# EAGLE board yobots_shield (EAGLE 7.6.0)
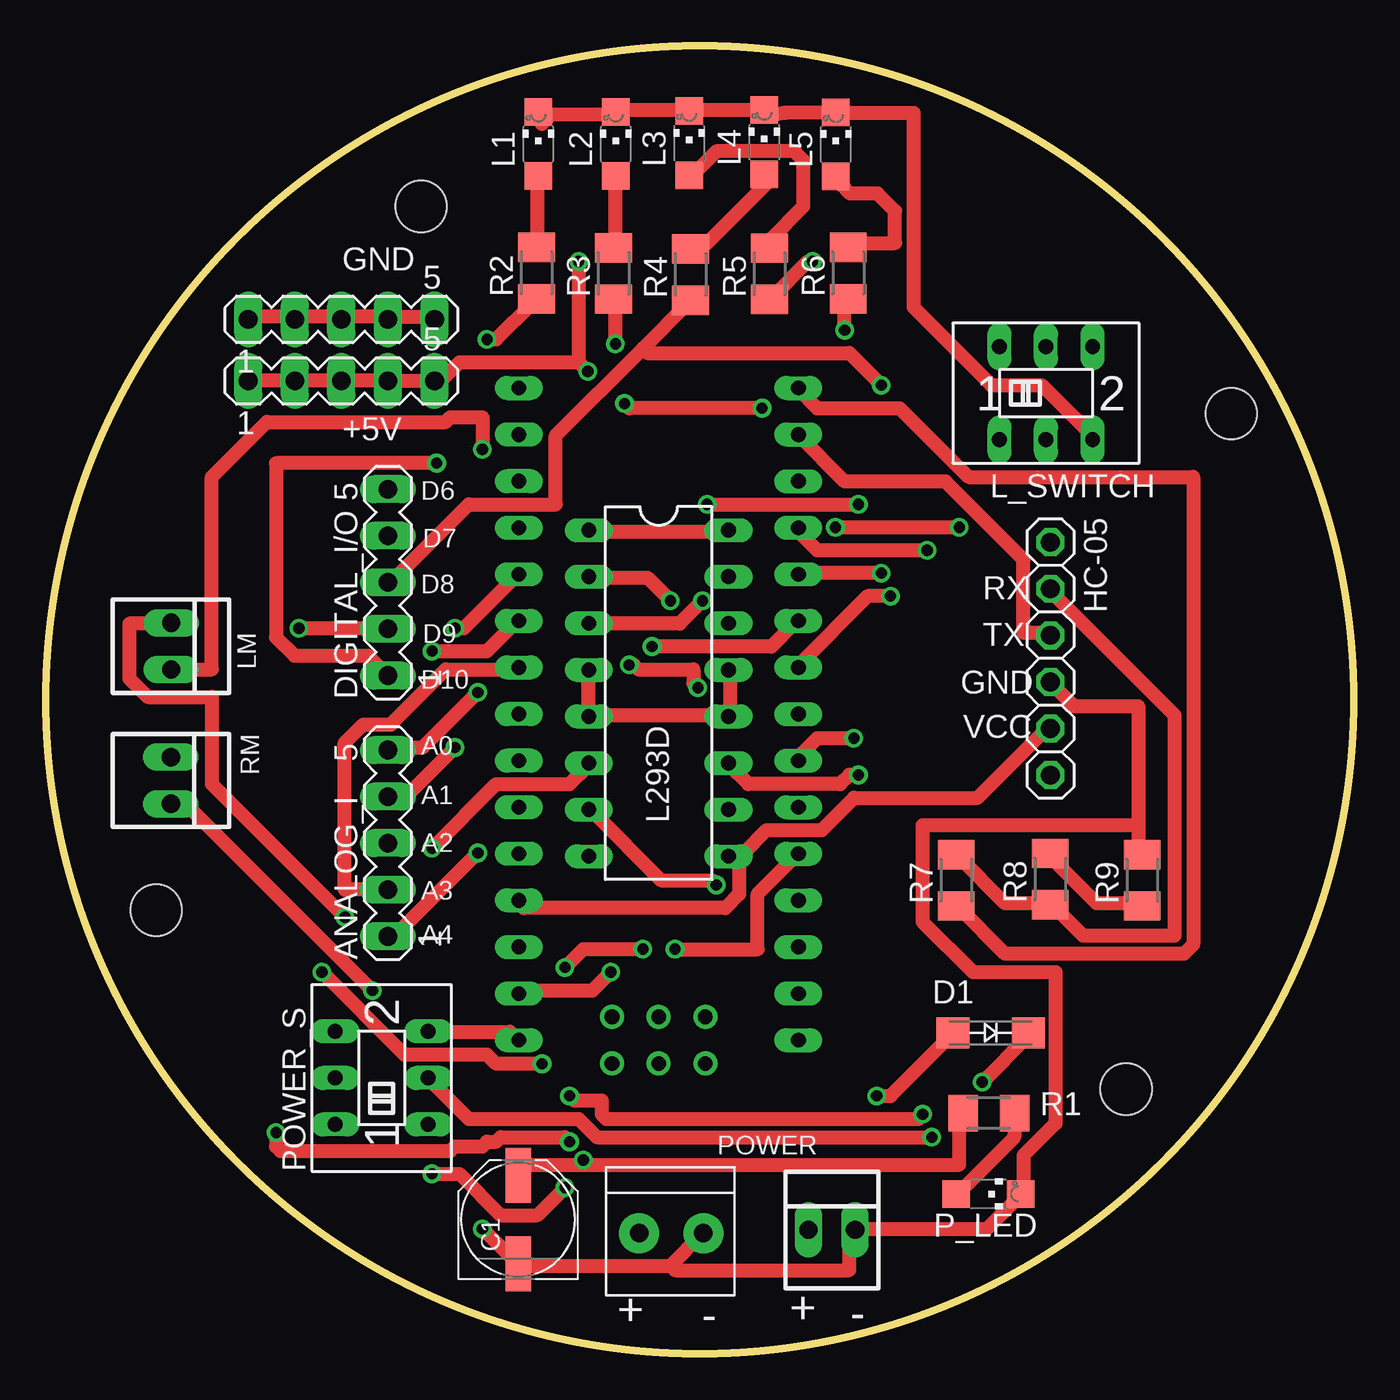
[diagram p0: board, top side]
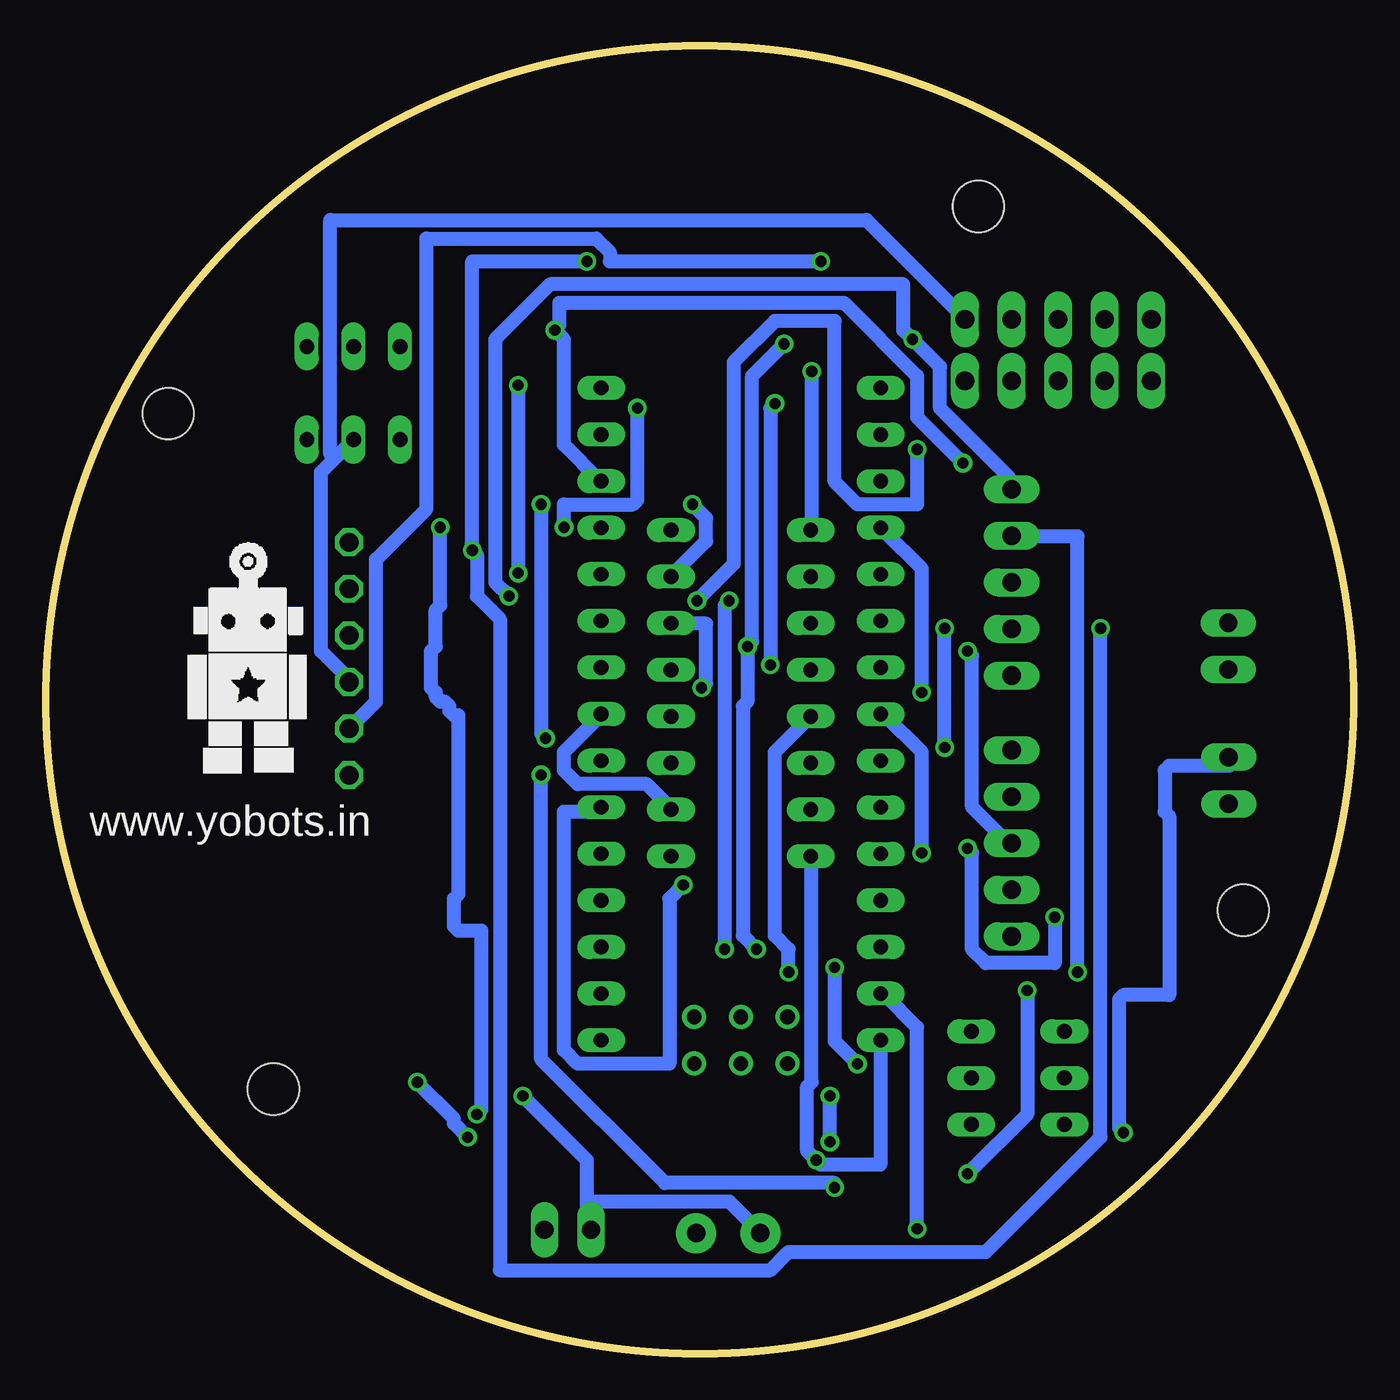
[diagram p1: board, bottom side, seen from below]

Size 71.3 x 71.3 mm. Coordinates in mm from the lower left corner, seen from the top.
Outline: circle at 35.65,35.65 radius 35.65
Copper layers (1*16): Top 0.035mm / dielectric 1.5mm / Bottom 0.035mm
Design rules "default": minimum track width 10mil, minimum drill 24mil, track to track 8mil, track to pad 8mil, pad to pad 8mil, via to via 8mil, smd to smd 8mil, copper to edge 40mil, drill to drill 8mil, minimum pad ring 10mil, minimum via ring 8mil, stop-mask expansion 4mil, vias tented up to drill 0mil, thermal gap 10mil
Net classes: 0 default: width 0.762 mm
Holes 2.8 mm at 20.45,62.55 64.63,51.25 58.9,14.42 6.01,24.18

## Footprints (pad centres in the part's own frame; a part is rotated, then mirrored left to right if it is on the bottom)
MA05-1 = drill 1.016 long: 1 -5.08,0; 2 -2.54,0; 3 0,0; 4 2.54,0; 5 5.08,0
PANASONIC_D = smd 3 x 1.4: + 2.4,0; - -2.4,0
SMA-DO214AC = smd 1.8 x 1.7: A -2.05,0; K 2.05,0
1X06 = drill 1.016 octagon: 1 -6.35,0; 2 -3.81,0; 3 -1.27,0; 4 1.27,0; 5 3.81,0; 6 6.35,0
1X2-3.5MM = drill 1 pad 2.184: 1 1.8,0; 2 -1.7,0
CHIPLED_1206 = smd 1.5 x 1.5: A 0,-1.75; C 0,1.75
DIL16 = drill 0.813 long: 1 -8.89,-3.81; 2 -6.35,-3.81; 3 -3.81,-3.81; 4 -1.27,-3.81; 5 1.27,-3.81; 6 3.81,-3.81; 7 6.35,-3.81; 8 8.89,-3.81; 9 8.89,3.81; 10 6.35,3.81; 11 3.81,3.81; 12 1.27,3.81; 13 -1.27,3.81; 14 -3.81,3.81; 15 -6.35,3.81; 16 -8.89,3.81
A68-A31 = drill 0.813 long: 1 -2.54,-2.54; 2 0,-2.54; 3 2.54,-2.54; 4 -2.54,2.54; 5 0,2.54; 6 2.54,2.54
22-23-2021 = drill 1 long: 1 -1.27,0; 2 1.27,0
M1206 = smd 1.6 x 2: 1 -1.4,0; 2 1.4,0
NANO = drill 0.8 long: 3.3V -10.16,24.13; 5V -10.16,-1.27; A0 -10.16,19.05; A1 -10.16,16.51; A2 -10.16,13.97; A3 -10.16,11.43; A4 -10.16,8.89; A5 -10.16,6.35; A6 -10.16,3.81; A7 -10.16,1.27; AREF -10.16,21.59; D2 5.08,1.27; D3 5.08,3.81; D4 5.08,6.35; D5 5.08,8.89; D6 5.08,11.43; D7 5.08,13.97; D8 5.08,16.51; D9 5.08,19.05; D10 5.08,21.59; D11 5.08,24.13; D12 5.08,26.67; D13 -10.16,26.67; GND -10.16,-6.35; GND1 5.08,-1.27; RAW -10.16,-8.89; RST -10.16,-3.81; RST1 5.08,-3.81; RX1 5.08,-6.35; TX0 5.08,-8.89 | drill 0.8: ICSP1 -5.08,-10.16; ICSP2 -5.08,-7.62; ICSP3 -2.54,-10.16; ICSP4 -2.54,-7.62; ICSP5 0,-10.16; ICSP6 0,-7.62

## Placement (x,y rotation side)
+5V  [MA05-1]  16.11,53.03 0 top
ANALOG_I  [MA05-1]  18.65,27.83 90 top
C1  [PANASONIC_D]  25.75,7.31 90 top
D1  [SMA-DO214AC]  51.51,17.49 0 top
DIGITAL_I/O  [MA05-1]  18.65,42.05 90 top
GND  [MA05-1]  16.11,56.39 0 top
HC-05  [1X06]  54.77,37.89 270 top
J1  [1X2-3.5MM]  34.15,6.57 180 top
L1  [CHIPLED_1206]  26.85,65.95 0 top
L2  [CHIPLED_1206]  31.07,65.95 0 top
L3  [CHIPLED_1206]  35.07,65.99 0 top
L4  [CHIPLED_1206]  39.17,66.05 0 top
L5  [CHIPLED_1206]  43.07,65.93 0 top
L293D  L293D  [DIL16]  33.41,36.01 270 top
L_SWITCH  [A68-A31]  54.53,52.37 0 top
LM  [22-23-2021]  6.83,38.57 270 top
P_LED  [CHIPLED_1206]  51.39,8.71 270 top
POWER  [22-23-2021]  42.85,6.75 0 top
POWER_S  [A68-A31]  18.31,15.03 90 top
R1  [M1206]  51.41,13.11 0 top
R2  [M1206]  26.75,58.91 90 top
R3  [M1206]  30.95,58.89 90 top
R4  [M1206]  35.15,58.83 90 top
R5  [M1206]  39.45,58.87 90 top
R6  [M1206]  43.75,58.91 90 top
R7  [M1206]  49.63,25.81 90 top
R8  [M1206]  54.75,25.87 90 top
R9  [M1206]  59.77,25.81 90 top
RM  [22-23-2021]  6.81,31.25 270 top
U$1  NANO  [NANO]  35.95,25.98 0 top

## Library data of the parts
+5V ANALOG_I DIGITAL_I/O GND = con-lstb; OC_FARNELL: unknown; OC_NEWARK: unknown
C1 = rcl
D1 = diode
HC-05 J1 L1-L5 P_LED R1-R9 = adafruit
L293D = st-microelectronics; MPN: L293D; OC_FARNELL: 9589619; OC_NEWARK: 56P8249
L_SWITCH POWER_S = switch
LM POWER RM = con-molex; MF: MOLEX; MPN: 22-23-2021; OC_FARNELL: 1462926; OC_NEWARK: 25C3832
U$1 = Arduino-clone

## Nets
5V: +5V.1 +5V.2 +5V.3 +5V.4 +5V.5 HC-05.5 L293D.1 L293D.9 L293D.16 U$1.5V
+9V: C1.+ L293D.8 POWER_S.3 R1.1 U$1.RAW
A0: ANALOG_I.5 U$1.A0
A1: ANALOG_I.4 U$1.A1
A2: ANALOG_I.3 U$1.A2
A3: ANALOG_I.2 U$1.A3
A4: ANALOG_I.1 U$1.A4
D2: L293D.2 U$1.D2
D3: L293D.7 U$1.D3
D4: L293D.15 U$1.D4
D5: L293D.10 U$1.D5
D6: DIGITAL_I/O.5 R2.1 U$1.D6
D7: DIGITAL_I/O.4 R3.1 U$1.D7
D8: DIGITAL_I/O.3 R4.1 U$1.D8
D9: DIGITAL_I/O.2 R5.1 U$1.D9
D10: DIGITAL_I/O.1 R6.1 U$1.D10
GND: C1.- GND.1 GND.2 GND.3 GND.4 GND.5 HC-05.4 J1.2 L293D.4 L293D.5 L293D.12 L293D.13 L_SWITCH.2 P_LED.C POWER.2 R9.2 U$1.GND
M1: L293D.3 LM.2
M2: L293D.6 LM.1
M3: L293D.14 RM.1
M4: L293D.11 RM.2
N$1: D1.A J1.1 POWER.1
N$2: P_LED.A R1.2
N$3: D1.K POWER_S.2
N$4: L1.A R2.2
N$5: L2.A R3.2
N$6: L4.A R4.2
N$7: HC-05.2 R7.2 R8.1
N$8: R8.2 R9.1
N$12: L3.A R5.2
N$13: L5.A R6.2
N$15: L1.C L2.C L3.C L4.C L5.C L_SWITCH.3
RX: HC-05.3 U$1.D11
TX: R7.1 U$1.D12

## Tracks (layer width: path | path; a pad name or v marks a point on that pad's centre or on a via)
5V  (via drill 0.61)
  Top 0.762: L293D.1 29.8,44.8 37.05,44.8 L293D.16 | +5V.1 11.05,53.05 13.55,53.05 +5V.2 13.8,53.05 15.8,53.05 +5V.3 16.3,53.05 18.55,53.05 +5V.4 18.8,53.05 21.05,53.05 +5V.5 21.55,53.05 22.55,54.05 29.05,54.05 | 29.05,54.05 v29.55,53.55 | U$1.5V 25.8,24.55 26.05,24.3 37.05,24.3 37.8,25.05 37.8,27.05 37.3,27.05 L293D.9 38.05,27.3 39.3,28.55 42.3,28.55 44.05,30.3 50.8,30.3 54.55,34.05 HC-05.5 | v29.05,59.55 29.05,54.05
  Bottom 0.762: v29.55,53.55 29.55,45.05 L293D.1 | v29.05,59.55 40.55,59.55 40.55,60.05 41.3,60.8 50.55,60.8 50.55,46.05 53.3,43.3 53.3,35.55 HC-05.5
+9V  (via drill 0.61)
  Top 0.762: U$1.RAW 25.55,17.3 25.3,17.55 21.05,17.55 POWER_S.3 | 29.3,10.3 26.3,10.3 25.8,9.8 C1.+ | 29.3,10.3 49.8,10.3 49.8,13.05 R1.1 | v29.3,10.55 29.3,10.3
  Bottom 0.762: L293D.8 29.55,27.05 29.55,14.8 29.8,14.55 29.8,11.05 v29.3,10.55 29.05,10.3 25.8,10.3 25.8,17.05 U$1.RAW
A0  (via drill 0.61)
  Top 0.762: v23.55,36.05 20.55,33.05 18.8,33.05 ANALOG_I.5
  Bottom 0.762: v23.55,36.05 23.55,42.8 25.55,44.8 U$1.A0
A1  (via drill 0.61)
  Top 0.762: v22.3,39.55 22.8,39.55 25.55,42.3 U$1.A1 | v22.3,33.05 19.8,30.55 18.8,30.55 ANALOG_I.4
  Bottom 0.762: v22.3,33.05 v22.3,39.55
A2  (via drill 0.61)
  Top 0.762: v21.05,38.3 24.05,38.3 25.55,39.8 U$1.A2
  Bottom 0.762: v21.05,38.3 20.8,38.05 20.8,29.8 18.8,27.8 ANALOG_I.3
A3
  Top 0.762: U$1.A3 25.55,37.3 21.8,37.3 18.8,34.3 17.3,34.3 16.3,33.3 16.3,25.3 18.55,25.3 ANALOG_I.2
A4  (via drill 0.61)
  Top 0.762: v23.55,27.3 19.05,22.8 18.8,22.8 ANALOG_I.1
  Bottom 0.762: v23.55,27.3 23.55,32.8 25.55,34.8 U$1.A4
D2  (via drill 0.61)
  Top 0.762: v34.3,22.05 38.8,22.05 38.8,25.05 40.8,27.05 U$1.D2 | v34.05,41.05 32.8,42.3 29.8,42.3 L293D.2
  Bottom 0.762: v34.3,22.05 34.3,40.8 v34.05,41.05
D3  (via drill 0.61)
  Top 0.762: v36.55,25.55 36.3,25.8 33.55,25.8 29.8,29.55 L293D.7
  Bottom 0.762: v36.55,25.55 37.3,24.8 37.3,15.8 42.3,15.8 43.05,16.55 43.05,29.55 41.05,29.55 U$1.D3
D4  (via drill 0.61)
  Top 0.762: v44.05,33.55 42.05,33.55 41.05,32.55 U$1.D4 | v36.05,46.3 v44.3,46.3
  Bottom 0.762: v44.05,33.55 44.3,33.8 v44.3,46.3 | v36.05,46.3 35.3,45.55 35.3,44.3 37.05,42.55 L293D.15
D5
  Bottom 0.762: U$1.D5 41.05,34.8 43.05,32.8 43.05,31.8 42.3,31.05 38.55,31.05 37.3,29.8 L293D.10
D6  (via drill 0.61)
  Top 0.762: v24.05,55.3 24.55,55.3 26.55,57.3 R2.1 | v46.05,41.3 44.8,41.3 41.05,37.55 U$1.D6
  Bottom 0.762: DIGITAL_I/O.5 18.8,47.3 18.8,47.8 22.55,51.55 22.55,53.8 v24.05,55.3 24.55,55.8 24.55,58.3 43.8,58.3 46.8,55.3 46.8,42.05 v46.05,41.3
D7  (via drill 0.61)
  Top 0.762: v31.05,55.05 31.05,57.3 R3.1 | v33.05,38.55 39.55,38.55 40.8,39.8 U$1.D7 | v15.05,20.8 19.55,16.3 24.05,16.3 24.55,15.8 v27.05,15.8 | v28.3,21.05 29.3,22.05 v32.55,22.05
  Bottom 0.762: v31.05,55.05 32.8,53.3 32.8,38.8 v33.05,38.55 33.05,35.55 33.3,35.3 33.3,22.8 v32.55,22.05 | v15.05,20.8 15.05,44.55 18.55,44.55 DIGITAL_I/O.4 | v27.05,15.8 28.3,17.05 v28.3,21.05
D8  (via drill 0.61)
  Top 0.762: 32.55,54.8 27.8,50.05 27.8,46.3 23.05,46.3 18.8,42.05 DIGITAL_I/O.3 | 32.55,54.8 35.05,57.3 R4.1 | v45.55,42.55 41.05,42.55 U$1.D8 | v45.55,52.8 43.8,54.55 32.8,54.55 32.55,54.8
  Bottom 0.762: v45.55,52.8 v45.55,42.55
D9  (via drill 0.61)
  Top 0.762: v41.8,59.55 41.55,59.55 39.55,57.55 R5.1 | v48.05,43.8 42.05,43.8 41.05,44.8 U$1.D9 | v13.8,39.55 18.55,39.55 DIGITAL_I/O.2
  Bottom 0.762: v41.8,59.55 48.05,59.55 v48.05,43.8 47.8,43.55 47.8,41.3 46.55,40.05 46.55,4.55 31.8,4.55 30.8,5.55 20.05,5.55 13.8,11.8 v13.8,39.55
D10  (via drill 0.61)
  Top 0.762: v43.55,55.8 43.55,57.3 R6.1 | v21.3,48.55 12.55,48.55 12.55,39.05 13.55,38.05 17.55,38.05 18.55,37.05 DIGITAL_I/O.1
  Bottom 0.762: U$1.D10 41.05,47.55 43.05,49.55 43.05,55.3 v43.55,55.8 43.3,56.05 43.3,57.3 27.8,57.3 23.8,53.3 23.8,51.05 v21.3,48.55
GND  (via drill 0.61)
  Top 0.762: L293D.4 29.55,37.05 29.55,34.8 L293D.5 29.8,34.8 37.05,34.8 L293D.12 37.3,34.8 37.3,37.05 L293D.13 | v23.8,6.8 25.55,5.05 C1.- 26.05,4.8 34.05,4.8 | 34.05,4.8 35.8,6.55 J1.2 | 34.05,4.8 34.3,4.55 43.8,4.55 43.8,6.55 POWER.2 44.3,6.8 51.3,6.8 53.05,8.55 P_LED.C 53.3,9.05 53.3,10.8 55.05,12.55 55.05,20.8 50.55,20.8 47.8,23.55 47.8,28.8 59.55,28.8 | v30.8,20.8 29.8,19.8 25.8,19.8 U$1.GND | GND.1 11.05,56.55 13.55,56.55 GND.2 13.8,56.55 15.8,56.55 GND.3 16.3,56.55 18.55,56.55 GND.4 18.8,56.55 21.05,56.55 GND.5 | 59.55,28.8 59.55,35.3 56.05,35.3 54.8,36.55 HC-05.4 | 59.55,28.8 59.55,27.3 R9.2
  Bottom 0.762: v23.8,6.8 23.8,17.8 25.55,19.55 U$1.GND | v30.8,20.8 30.8,22.05 31.55,22.8 31.55,32.8 29.8,34.55 L293D.5 | 55.55,48.8 56.3,48.05 56.3,38.3 54.8,36.8 HC-05.4 | 55.55,48.8 54.55,49.8 L_SWITCH.2 | GND.5 21.3,56.55 26.55,61.8 55.8,61.8 55.8,49.05 55.55,48.8
M1  (via drill 0.61)
  Top 0.762: v35.8,41.05 34.55,39.8 29.8,39.8 L293D.3 | v23.8,49.3 23.8,51.05 22.05,51.05 21.8,50.8 12.05,50.8 9.05,47.8 9.05,37.3 LM.2
  Bottom 0.762: v35.8,41.05 33.8,43.05 33.8,54.05 31.55,56.3 28.3,56.3 28.3,47.55 27.05,46.3 23.8,46.3 v23.8,49.3
M2  (via drill 0.61)
  Top 0.762: v21.05,27.55 24.55,31.05 28.55,31.05 29.55,32.05 L293D.6 | v16.3,23.8 9.05,31.05 9.05,35.8 5.55,35.8 4.55,36.8 4.55,39.8 6.8,39.8 LM.1
  Bottom 0.762: v21.05,27.55 20.8,27.3 20.8,22.05 20.05,21.3 16.3,21.3 v16.3,23.8
M3  (via drill 0.61)
  Top 0.762: v35.55,36.3 35.3,36.55 35.3,37.3 32.3,37.3 32.05,37.55 v31.8,37.55 | v31.55,51.8 31.8,51.55 v39.05,51.55 | v49.8,45.05 v43.05,45.05 | v47.8,13.05 47.55,12.8 30.55,12.8 30.3,13.05 30.3,13.8 28.8,13.8 v28.55,14.05 | v28.55,11.55 28.3,11.8 24.8,11.8 24.55,11.55 24.05,11.55 23.8,11.3 22.3,11.3 22.05,11.05 12.8,11.05 12.55,11.3 v12.55,12.05
  Bottom 0.762: v35.55,36.3 35.3,36.55 35.3,39.8 37.05,39.8 L293D.14 | v31.8,37.55 31.8,51.55 v31.55,51.8 | v39.05,51.55 39.05,46.55 39.3,46.3 43.05,46.3 v43.05,45.05 | v49.8,45.05 49.8,40.8 50.05,40.55 50.05,38.55 50.3,38.3 50.3,36.3 50.05,36.05 50.05,35.8 49.8,35.55 49.55,35.55 49.3,35.3 49.3,35.05 49.05,34.8 48.8,34.8 48.8,25.05 49.05,24.8 49.05,23.3 48.8,23.05 47.55,23.05 47.55,13.3 v47.8,13.05 | v28.55,11.55 v28.55,14.05 | v12.55,12.05 12.8,12.3 12.8,19.3 12.55,19.55 10.05,19.55 10.05,29.3 10.3,29.55 10.3,31.8 10.05,32.05 6.8,32.05 6.8,32.3 RM.1
M4  (via drill 0.61)
  Top 0.762: v44.3,31.55 43.8,31.55 43.3,31.05 38.3,31.05 37.3,32.05 L293D.11 | v28.3,9.05 26.8,7.55 24.8,7.55 22.55,9.8 v21.05,9.8 | v17.8,19.8 7.8,29.8 7.05,29.8 RM.2
  Bottom 0.762: v44.3,31.55 44.3,16.05 37.55,9.3 28.3,9.3 v28.3,9.05 | v21.05,9.8 17.8,13.05 v17.8,19.8
N$1  (via drill 0.61)
  Top 0.762: v45.3,14.05 46.05,14.05 49.3,17.3 D1.A
  Bottom 0.762: v45.3,14.05 41.8,10.55 41.8,8.3 | 41.8,8.3 41.8,6.8 POWER.1 | 41.8,8.3 34.05,8.3 32.55,6.8 J1.1
N$2
  Top 0.762: P_LED.A 49.8,8.8 52.8,11.8 52.8,13.05 R1.2
N$3  (via drill 0.61)
  Top 0.762: v51.05,14.8 53.55,17.3 D1.K | v48.3,11.8 30.05,11.8 29.05,12.8 23.05,12.8 21.05,14.8 POWER_S.2
  Bottom 0.762: v51.05,14.8 49.05,12.8 49.05,12.55 v48.3,11.8
N$4
  Top 0.762: L1.A 26.8,63.3 26.8,60.55 R2.2
N$5
  Top 0.762: L2.A 31.05,64.05 31.05,60.3 R3.2
N$6
  Top 0.762: L4.A 39.55,64.05 35.8,60.3 35.3,60.3 R4.2
N$7
  Top 0.762: R7.2 49.8,27.05 52.3,24.55 54.55,24.55 R8.1 55.05,24.3 56.55,22.8 61.55,22.8 61.55,34.8 54.8,41.55 HC-05.2
N$8
  Top 0.762: R8.2 54.8,27.05 57.3,24.55 59.55,24.55 R9.1
N$12
  Top 0.762: L3.A 35.55,64.55 36.55,65.55 40.8,65.55 41.3,65.05 41.3,62.55 39.55,60.8 39.55,60.3 R5.2
N$13
  Top 0.762: L5.A 43.4,63.7 43.85,63.25 45.35,63.25 46.3,62.3 46.3,60.55 43.8,60.55 R6.2
N$15
  Top 0.762: L1.C 27.05,67.05 27.55,67.55 31.05,67.55 L2.C 31.3,67.8 35.3,67.8 L3.C 35.55,67.8 L4.C | L4.C 39.8,67.55 40.3,67.65 43.55,67.65 L5.C 43.8,67.65 47.3,67.65 47.3,57.05 51.55,52.8 54.3,52.8 57.05,50.05 L_SWITCH.3 | 39.55,67.8 L4.C
RX
  Top 0.762: U$1.D11 41.05,50.05 43.55,47.55 49.05,47.55 53.3,43.3 53.3,39.3 54.55,39.3 HC-05.3
TX
  Top 0.762: R7.1 49.8,24.3 52.3,21.8 62.05,21.8 62.55,22.3 62.55,47.8 50.3,47.8 46.55,51.55 42.05,51.55 41.05,52.55 U$1.D12

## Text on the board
tNames: D6 | D7 | D8 | RX | D9 | TX | D10 | GND | VCC | A0 | A1 | A2 | A3 | A4 | + | - | + | -
bNames: www.yobots.in | E:/yobots/yobots logo 10mmx10mm - Copy.bmp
